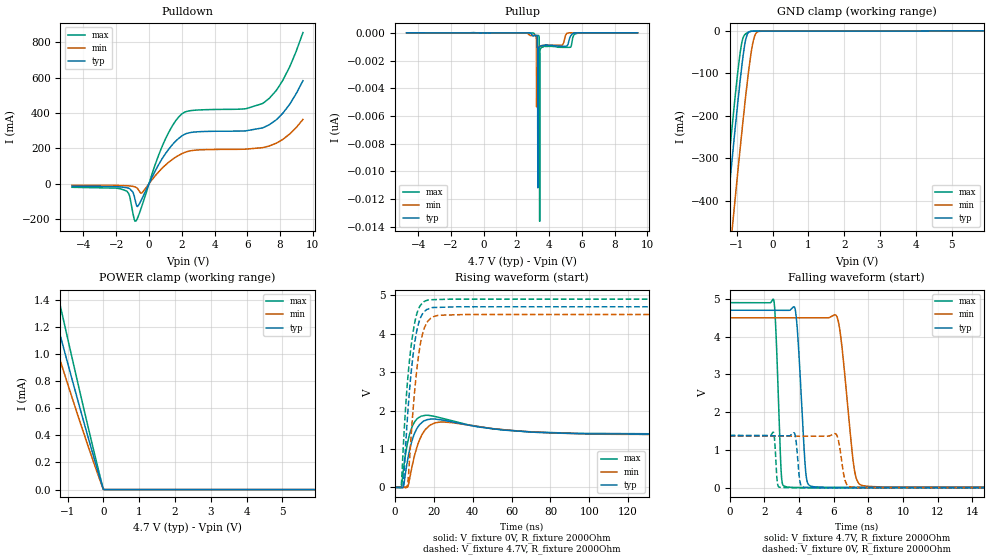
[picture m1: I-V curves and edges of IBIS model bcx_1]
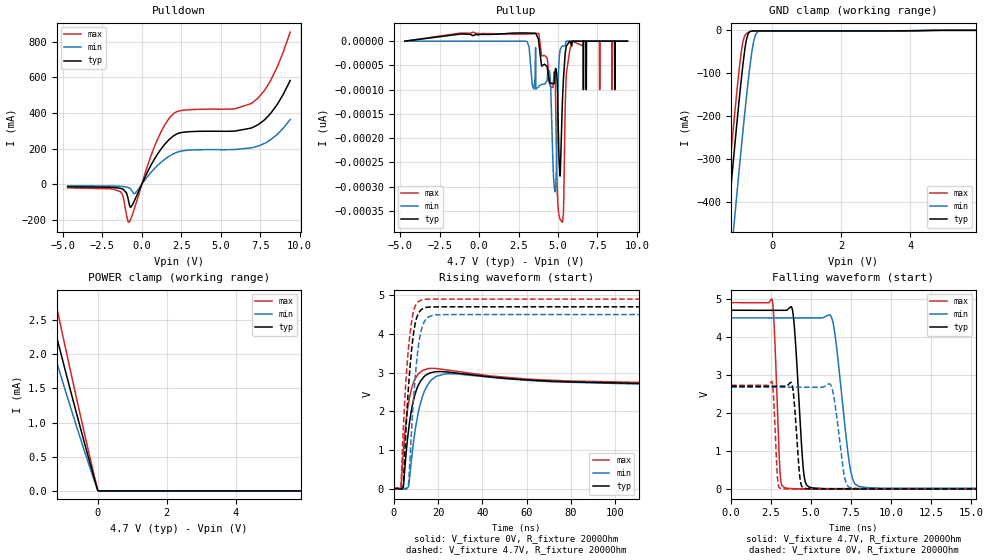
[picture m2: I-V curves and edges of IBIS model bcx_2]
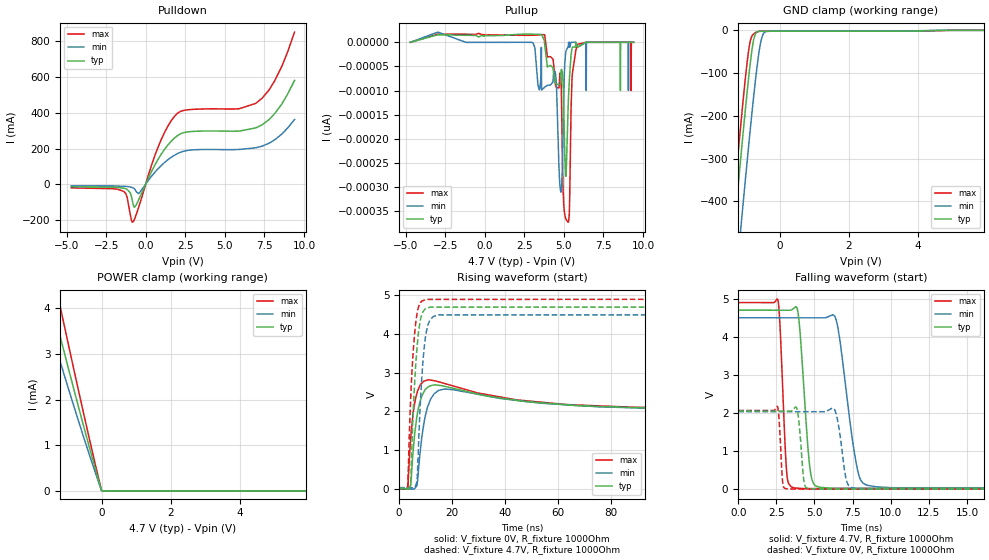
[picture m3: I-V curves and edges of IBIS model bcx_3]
| Texas Instruments Incorporated
| TPS546D24A- 2.95V to 16V, 40A, up to 4X stackable, PMBus(R) buck converter
| Marketing part#   Digital Voltage Range   Package-type   #pins
| TPS546D24A   0V - 5.5V   LQFN-CLIP   40
[IBIS Ver]   4.1
[File name]   tps546d24a.ibs
[File Rev]   1.0
[Date]   11/21/2019
[Source]
| Texas Instruments Incorporated.
| Analog-eLab Design Center, HPA
| 12500 TI Blvd
| Dallas, TX -75243
[Notes]   Revision History:
| Rev 1.0: 11/21/2019
| - Initial version of the model
| - Model generated from simulations in SPECTRE
| - C_comp although listed in numerical order of value are
|   obtained from varying PVT conditions. For PVT conditions for
|   each specific value refer the buffer description under
|   respective [Model]. IBIS model user is responsible for using
|   appropriate C_comp to simulate for Signal Integrity.
| - Warnings regarding combined Non-monotonicity of various models have been
|   reviewed and considered minor and can be ignored.
| - Model names with a trailing _1p8 contain the model for 1.8V operation.
|   Model names with a trailing _2p5 contain the model for 2.5V operation.
|   Model names with a trailing _3p3 contain the model for 3.3V operation.
|   Model names with a trailing _5p0 contain the model for 5.0V operation.
[Disclaimer]
| This model is designed as an aid for customers of Texas Instruments.
| TI and its licensors and suppliers make no warranties, either expressed
| or implied, with respect to this  model, including the warranties of
| merchantability or fitness for a particular purpose. The model is
| provided solely on an "as is" basis. The entire risk as to its quality
| and performance is with the customer.
| This model is subject to change without notice. Texas Instruments
| Incorporated is not responsible for updating this model
[Copyright]
(C) Copyright 2019 Texas Instruments Incorporated.All rights reserved.
|  Component TPS546D24RVF 40-Pin LQFN-CLIP -RVF package
|  Part # TPS546D24RVF
[Component]   TPS546D24RVF
[Manufacturer]   TI
[Package]   |40 LQFN-CLIP -RVF package
|   typ   min   max
R_pkg   0.05   0.04   0.06
L_pkg   1.0nH   0.8nH   1.2nH
C_pkg   0.2pF   0.16pF   0.24pF
[Pin] signal_name  model_name   R_pin   L_pin   C_pin
1   PGD/RST_B   pgd   NA   NA   NA
2   PMB_DATA   pmb   NA   NA   NA
3   PMB_CLK   pmb   NA   NA   NA
4   BP1V5   nc   NA   NA   NA
5   DRTN   nc   NA   NA   NA
6   SMB_ALRT   pmb   NA   NA   NA
7   BOOT   nc   NA   NA   NA
8   SW   nc   NA   NA   NA
9   SW   nc   NA   NA   NA
10   SW   nc   NA   NA   NA
11   SW   nc   NA   NA   NA
12   SW   nc   NA   NA   NA
13   PGND   gnd   NA   NA   NA
14   PGND   gnd   NA   NA   NA
15   PGND   gnd   NA   NA   NA
16   PGND   gnd   NA   NA   NA
17   PGND   gnd   NA   NA   NA
18   PGND   gnd   NA   NA   NA
19   PGND   gnd   NA   NA   NA
20   PGND   gnd   NA   NA   NA
21   PVIN   power   NA   NA   NA
22   PVIN   power   NA   NA   NA
23   PVIN   power   NA   NA   NA
24   PVIN   power   NA   NA   NA
25   PVIN   power   NA   NA   NA
26   AVIN   power   NA   NA   NA
27   EN/UVLO   nc   NA   NA   NA
28   VDD5   power   NA   NA   NA
29   MSEL2   nc   NA   NA   NA
30   VSEL   nc   NA   NA   NA
31   ADRSEL   nc   NA   NA   NA
32   MSEL1   nc   NA   NA   NA
33   VOSNS   nc   NA   NA   NA
34   GOSNS/SLAVE   nc   NA   NA   NA
35   VSHARE   nc   NA   NA   NA
36   NC   nc   NA   NA   NA
37   AGND   gnd   NA   NA   NA
38   SYNC   sync   NA   NA   NA
39   BCX_CLK   bcx   NA   NA   NA
40   BCX_DAT   bcx   NA   NA   NA
|   Model Selectors
[Model Selector] pmb
pmb_1p8   1.8V   Digital I/O
pmb_2p5   2.5V   Digital I/O
pmb_3p3   3.3V   Digital I/O
pmb_5p0   5.0V   Digital I/O
[Model Selector] bcx
bcx_1   One Pullup Current source block(672uA)   Digital I/O | 672uA constant pullup current
bcx_2   Two Pullup Current source blocks(2*672uA   Digital I/O | 1.34mA constant pullup current
bcx_3   Three Pullup Current source blocks(3*672uA)  Digital I/O | 2mA constant pullup current
| Models and submodels in the file (9): bcx_1 (I/O), bcx_2 (I/O), bcx_3 (I/O), pmb_1p8 (I/O_open_drain), pmb_2p5 (I/O_open_drain), pmb_3p3 (I/O_open_drain), pmb_5p0 (I/O_open_drain), pgd (I/O_open_drain), sync (I/O)
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|   bcx_1 Model
[Model]   bcx_1
Model_type   I/O
Polarity   Inverting
Enable   Active-High
Vinl = 0.8
Vinh = 1.35
Vmeas = 2.35
Vref = 0
Cref = 2pF
Rref = 100000
|   typ   min   max
C_comp   2.976pF   2.962pF   2.990pF
|C_comp_pull_up   2.976pF   2.962pF   2.990pF
|C_comp_pull_down   3.370pF   3.218pF   3.645pF
|  Where Nom  PVT is Nominal Process, 4.7V,  25C
|   Fast PVT is Strong Process,  4.9V,  -40C
|   Slow PVT is Weak Process,   4.5V,  150C
[Voltage Range]   4.7   4.5   4.9
|Junction Temperature
[Temperature Range]   25   150   -40
[Pullup Reference]   4.7   4.5   4.9
[Pulldown Reference]   0   0   0
[Power Clamp Reference]   4.7   4.5   4.9
[GND Clamp Reference]   0   0   0
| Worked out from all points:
|   slope of the pulldown table from 0 to 0.705 V, typ, clamps not added: 5.58 ohm
|   GND clamp passes 1 mA (typ) near -0.59 V on its own axis
|   POWER clamp passes 1 mA (typ) near -1.07 V on its own axis
|   falling waveform, V_fixture 4.7V, R_fixture 2000Ohm: 20-80 % time 340ps typ, 567ps min, 230ps max; typ from 4.7 V to 0.009 V
|   rising waveform, V_fixture 0V, R_fixture 2000Ohm: 20-80 % time 3.01ns typ, 3.88ns min, 2.35ns max; typ from 0 V to 1.38 V
|   rising waveform, V_fixture 4.7V, R_fixture 2000Ohm: 20-80 % time 4.82ns typ, 4.91ns min, 4.75ns max; typ from 0.009 V to 4.7 V
|   falling waveform, V_fixture 0V, R_fixture 2000Ohm: 20-80 % time 159ps typ, 276ps min, 104ps max; typ from 1.38 V to 0 V
[Pulldown]
|   Voltage   I(typ)   I(min)   I(max)
-4.7V     -13.03mA   -7.807mA   -19.31mA
-1.372V   -21.4mA    -10.46mA   -39.93mA
-1.175V   -27.33mA   -11.73mA   -70.85mA
-977.6mV  -47.06mA   -14.22mA   -167.8mA
-780.2mV  -116.5mA   -20.57mA   -208.3mA
-441.8mV  -86.15mA   -51.84mA   -127.7mA
799mV     141.5mA    88.06mA    211mA
1.786V    255.1mA    159.9mA    375.5mA
2.378V    287.2mA    183.7mA    411.3mA
7.003V    319.1mA    206.2mA    458.6mA
8.173V    399.9mA    251.8mA    586.2mA
9.4V      583.6mA    364.2mA    855.5mA
[GND Clamp]
|   Voltage   I(typ)   I(min)   I(max)
-4.7V     -3.614A    -3.753A    -3.556A
-1.415V   -552.2mA   -718.1mA   -475.4mA
-1.387V   -526.9mA   -693mA     -450mA
-1.358V   -501.7mA   -667.9mA   -424.6mA
-1.175V   -339.6mA   -506.1mA   -262.5mA
-1.076V   -254.6mA   -420.3mA   -178.5mA
-864.8mV  -85.71mA   -242.2mA   -29.58mA
-752mV    -20.4mA    -153.3mA   -6.976mA
-667.4mV  -3.13mA    -92.52mA   -2.572mA
-540.5mV  -779.1uA   -23.54mA   -798uA
-385.4mV  -692.5uA   -1.346mA   -696.8uA
9.4V      0A         0A         0A
[Pullup]
|   Voltage   I(typ)   I(min)   I(max)
-4.7V     0A         0A         0A
3.238V    -198.4pA   -5.351nA   -223.5pA
3.252V    -214.7pA   -1.335nA   -215.3pA
3.295V    -1.813nA   -1.09nA    -192.7pA
3.309V    -11.18nA   -1.068nA   -191.3pA
3.323V    -1.223nA   -1.048nA   -185.8pA
3.365V    -1.077nA   -1.002nA   -208.2pA
3.408V    -1.009nA   -972.6pA   -2.075nA
3.422V    -994.3pA   -965pA     -13.59nA
3.436V    -981.8pA   -958.2pA   -1.319nA
3.478V    -955.2pA   -942.1pA   -1.14nA
9.4V      0A         0A         0A
[POWER Clamp]
|   Voltage   I(typ)   I(min)   I(max)
-4.7V     4.841mA    4.462mA    5.649mA
-1.852V   1.785mA    1.503mA    2.128mA
-1.683V   1.613mA    1.356mA    1.924mA
-1.528V   1.457mA    1.223mA    1.739mA
-1.175V   1.106mA    925.7uA    1.321mA
-709.7mV  653.4uA    544.2uA    781.1uA
-314.9mV  282.1uA    233.9uA    337.5uA
-4.7mV    3.975uA    3.346uA    4.745uA
23.5mV    0A         0A         0A
9.4V      0A         0A         0A
[Ramp]
R_load = 2000
|   typ   min   max
dV/dt_r   0.827359/3.01437e-09   0.821238/3.8948e-09   0.83293/2.35068e-09
dV/dt_f   2.81451/3.39702e-10   2.69064/5.67144e-10   2.93668/2.30357e-10
[Falling Waveform]
V_fixture = 4.7V
V_fixture_min = 4.5V
V_fixture_max = 4.9V
R_fixture = 2000Ohm
C_fixture = 0F
|   Time   V(typ)   V(min)   V(max)
0s        4.7V       4.5V       4.9V
2.532ns   4.698V     4.499V     4.99V
3.009ns   4.698V     4.499V     209.5mV
3.791ns   4.697V     4.498V     9.359mV
4.45ns    212mV      4.498V     9.354mV
5.517ns   13.54mV    4.498V     9.346mV
6.303ns   13.53mV    4.331V     9.34mV
7.333ns   13.52mV    218.5mV    9.332mV
8.874ns   13.51mV    21.85mV    9.32mV
500ns     9.15mV     15.58mV    5.526mV
[Rising Waveform]
V_fixture = 0V
V_fixture_min = 0V
V_fixture_max = 0V
R_fixture = 2000Ohm
C_fixture = 0F
|   Time   V(typ)   V(min)   V(max)
0s        -2.427nV   5.037nV    271.9pV
3.238ns   656.8uV    388.6uV    -5.328mV
4.261ns   -190uV     511.4uV    444.5mV
6.531ns   731.8mV    13.27mV    1.18V
10ns      1.404V     824.6mV    1.699V
15.76ns   1.748V     1.516V     1.878V
24.37ns   1.754V     1.705V     1.798V
50.88ns   1.523V     1.527V     1.522V
91.31ns   1.404V     1.403V     1.41V
500ns     1.379V     1.369V     1.388V
[Rising Waveform]
V_fixture = 4.7V
V_fixture_min = 4.5V
V_fixture_max = 4.9V
R_fixture = 2000Ohm
C_fixture = 0F
|   Time   V(typ)   V(min)   V(max)
0s        9.15mV     15.58mV    5.526mV
3.185ns   9.792mV    10.32mV    27.19mV
4.261ns   67.08mV    8.545mV    1.075V
6.468ns   1.883V     67.45mV    2.788V
9.358ns   3.481V     2.076V     4.063V
11.85ns   4.221V     3.339V     4.619V
14.39ns   4.54V      4.041V     4.816V
17.2ns    4.647V     4.342V     4.879V
36.2ns    4.7V       4.5V       4.9V
500ns     4.7V       4.5V       4.9V
[Falling Waveform]
|Gnd
V_fixture = 0V
V_fixture_min = 0V
V_fixture_max = 0V
R_fixture = 2000Ohm
C_fixture = 0F
|   Time   V(typ)   V(min)   V(max)
0s        1.379V     1.369V     1.389V
2.523ns   1.377V     1.368V     1.474V
2.792ns   1.377V     1.368V     53.28mV
3.739ns   1.449V     1.367V     2.287mV
3.941ns   682.9mV    1.367V     1.025mV
4.174ns   33.24mV    1.367V     1.025mV
6.123ns   1.585mV    1.43V      1.021mV
6.773ns   1.583mV    82.23mV    1.02mV
8.526ns   1.577mV    2.589mV    1.016mV
500ns     -359.2pV   -5.119nV   309.4pV
|   bcx_2 Model
[Model]   bcx_2
Model_type   I/O
Polarity   Inverting
Enable   Active-High
Vinl = 0.8
Vinh = 1.35
Vmeas = 2.35
Vref = 0
Cref = 2pF
Rref = 100000
|   typ   min   max
C_comp   2.976pF   2.976pF   2.990pF
|C_comp_pull_up   2.976pF   2.962pF   2.977pF
|C_comp_pull_down   3.204pF   3.088pF   3.401pF
|  Where Nom  PVT is Nominal Process, 4.7V,  25C
|   Fast PVT is Strong Process,  4.9V,  -40C
|   Slow PVT is Weak Process,   4.5V,  150C
[Voltage Range]   4.7   4.5   4.9
|Junction Temperature
[Temperature Range]   25   150   -40
[Pullup Reference]   4.7   4.5   4.9
[Pulldown Reference]   0   0   0
[Power Clamp Reference]   4.7   4.5   4.9
[GND Clamp Reference]   0   0   0
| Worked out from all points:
|   slope of the pulldown table from 0 to 0.705 V, typ, clamps not added: 5.58 ohm
|   POWER clamp passes 1 mA (typ) near -0.55 V on its own axis
|   falling waveform, V_fixture 4.7V, R_fixture 2000Ohm: 20-80 % time 398ps typ, 688ps min, 264ps max; typ from 4.7 V to 0.009 V
|   rising waveform, V_fixture 0V, R_fixture 2000Ohm: 20-80 % time 3.4ns typ, 4.17ns min, 2.75ns max; typ from 0 V to 2.71 V
|   rising waveform, V_fixture 4.7V, R_fixture 2000Ohm: 20-80 % time 3.38ns typ, 3.49ns min, 3.27ns max; typ from 0.009 V to 4.7 V
|   falling waveform, V_fixture 0V, R_fixture 2000Ohm: 20-80 % time 278ps typ, 479ps min, 180ps max; typ from 2.71 V to 0 V
[Pulldown]
|   Voltage   I(typ)   I(min)   I(max)
-4.7V     -12.99mA   -7.762mA   -19.27mA
-1.372V   -21.32mA   -10.38mA   -39.86mA
-1.175V   -27.24mA   -11.64mA   -70.76mA
-977.6mV  -46.92mA   -14.12mA   -167.7mA
-780.2mV  -116.1mA   -20.42mA   -207.7mA
-441.8mV  -85.46mA   -51.2mA    -127mA
799mV     142.2mA    88.74mA    211.7mA
1.786V    255.8mA    160.6mA    376.2mA
2.576V    291.6mA    188.3mA    415.1mA
7.003V    318.3mA    205.9mA    457.3mA
8.173V    398.9mA    251.3mA    584.4mA
9.4V      582mA      363.3mA    852.9mA
[GND Clamp]
|   Voltage   I(typ)   I(min)   I(max)
-4.7V     -3.614A    -3.753A    -3.556A
-1.415V   -552.3mA   -718.2mA   -475.5mA
-1.387V   -527mA     -693mA     -450mA
-1.358V   -501.7mA   -667.9mA   -424.7mA
-1.175V   -339.7mA   -506.2mA   -262.6mA
-1.076V   -254.7mA   -420.4mA   -178.6mA
-864.8mV  -85.91mA   -242.3mA   -29.97mA
-766.1mV  -26.69mA   -164.2mA   -8.741mA
-667.4mV  -3.776mA   -92.75mA   -3.245mA
-540.5mV  -1.469mA   -23.98mA   -1.492mA
-385.4mV  -1.384mA   -2.021mA   -1.393mA
9.4V      0A         0A         0A
[Pullup]
|   Voltage   I(typ)   I(min)   I(max)
-4.7V     0A         0A         0A
3.788V    -5pA       -92.8pA    14.9pA
4.451V    -83.2pA    -60.9pA    -84.9pA
4.817V    -62.2pA    -310.8pA   -82.8pA
4.958V    -95.3pA    -162.3pA   -315.9pA
5.128V    -278.2pA   -20pA      -366.9pA
5.255V    -148.2pA   -10pA      -373.2pA
5.508V    -13pA      0A         -79.2pA
5.889V    0A         0A         0A
6.608V    -100pA     0A         0A
7.638V    0A         0A         -100pA
9.4V      0A         0A         0A
[POWER Clamp]
|   Voltage   I(typ)   I(min)   I(max)
-4.7V     9.671mA    8.914mA    11.28mA
-1.852V   3.566mA    3.004mA    4.25mA
-1.697V   3.252mA    2.735mA    3.878mA
-1.499V   2.855mA    2.396mA    3.406mA
-1.175V   2.211mA    1.85mA     2.64mA
-766.1mV  1.414mA    1.178mA    1.69mA
-371.3mV  667.9uA    554.2uA    798.7uA
-4.7mV    8.089uA    6.692uA    9.665uA
23.5mV    0A         0A         0A
9.4V      0A         0A         0A
[Ramp]
R_load = 2000
|   typ   min   max
dV/dt_r   1.62317/3.40511e-09   1.60666/4.16841e-09   1.63751/2.75863e-09
dV/dt_f   2.81451/3.97943e-10   2.69064/6.88264e-10   2.93668/2.64301e-10
[Falling Waveform]
V_fixture = 4.7V
V_fixture_min = 4.5V
V_fixture_max = 4.9V
R_fixture = 2000Ohm
C_fixture = 0F
|   Time   V(typ)   V(min)   V(max)
0s        4.7V       4.5V       4.9V
2.56ns    4.698V     4.499V     4.989V
3.119ns   4.698V     4.499V     196mV
3.79ns    4.777V     4.499V     14.95mV
4.035ns   3.817V     4.498V     9.15mV
4.698ns   133mV      4.498V     9.145mV
6.299ns   13.29mV    4.496V     9.134mV
7.657ns   13.28mV    210.8mV    9.124mV
9.53ns    13.27mV    20.93mV    9.11mV
500ns     9.15mV     15.58mV    5.526mV
[Rising Waveform]
V_fixture = 0V
V_fixture_min = 0V
V_fixture_max = 0V
R_fixture = 2000Ohm
C_fixture = 0F
|   Time   V(typ)   V(min)   V(max)
0s        -6.173nV   232pV      -228.1pV
3.229ns   -9.546mV   -5.91mV    24.76mV
4.326ns   53.39mV    -7.921mV   969.3mV
6.62ns    1.491V     55.89mV    2.2V
8.404ns   2.163V     969.4mV    2.66V
11ns      2.667V     1.956V     2.962V
15.46ns   2.965V     2.695V     3.103V
24.68ns   3.012V     2.972V     3.063V
109ns     2.725V     2.707V     2.75V
500ns     2.705V     2.678V     2.729V
[Rising Waveform]
V_fixture = 4.7V
V_fixture_min = 4.5V
V_fixture_max = 4.9V
R_fixture = 2000Ohm
C_fixture = 0F
|   Time   V(typ)   V(min)   V(max)
0s        9.15mV     15.58mV    5.526mV
3.214ns   9.757mV    10.61mV    48.23mV
4.326ns   116.9mV    8.884mV    1.582V
6.559ns   2.561V     100.2mV    3.585V
8.404ns   3.78V      1.874V     4.448V
10ns      4.351V     3.098V     4.761V
11.45ns   4.559V     3.818V     4.849V
13.25ns   4.655V     4.252V     4.888V
24.68ns   4.7V       4.5V       4.9V
500ns     4.7V       4.5V       4.9V
[Falling Waveform]
|Gnd
V_fixture = 0V
V_fixture_min = 0V
V_fixture_max = 0V
R_fixture = 2000Ohm
C_fixture = 0F
|   Time   V(typ)   V(min)   V(max)
0s        2.705V     2.678V     2.729V
2.545ns   2.704V     2.677V     2.83V
2.959ns   2.703V     2.677V     100.4mV
3.917ns   2.436V     2.676V     2.259mV
4.275ns   423.8mV    2.676V     2.257mV
4.464ns   48.14mV    2.676V     2.257mV
6.201ns   3.489mV    2.756V     2.249mV
7.23ns    3.482mV    131.6mV    2.244mV
8.973ns   3.47mV     3.468mV    2.236mV
500ns     -610.1pV   7.057nV    1.367nV
|   bcx_3 Model
[Model]   bcx_3
Model_type   I/O
Polarity   Inverting
Enable   Active-High
Vinl = 0.8
Vinh = 1.35
Vmeas = 2.35
Vref = 0
Cref = 2pF
Rref = 100000
|   typ   min   max
C_comp   2.990pF   2.976pF   2.990pF
|C_comp_pull_up   2.977pF   2.976pF   2.990pF
|C_comp_pull_down   3.189pF   3.116pF   3.324pF
|  Where Nom  PVT is Nominal Process, 4.7V,  25C
|   Fast PVT is Strong Process,  4.9V,  -40C
|   Slow PVT is Weak Process,   4.5V,  150C
[Voltage Range]   4.7   4.5   4.9
|Junction Temperature
[Temperature Range]   25   150   -40
[Pullup Reference]   4.7   4.5   4.9
[Pulldown Reference]   -0   0   0
[Power Clamp Reference]   4.7   4.5   4.9
[GND Clamp Reference]   0   0   0
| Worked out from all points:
|   slope of the pulldown table from 0 to 0.705 V, typ, clamps not added: 5.58 ohm
|   POWER clamp passes 1 mA (typ) near -0.37 V on its own axis
|   falling waveform, V_fixture 4.7V, R_fixture 1000Ohm: 20-80 % time 481ps typ, 864ps min, 310ps max; typ from 4.7 V to 0.018 V
|   rising waveform, V_fixture 0V, R_fixture 1000Ohm: 20-80 % time 1.58ns typ, 2ns min, 1.25ns max; typ from 0 V to 2.05 V
|   rising waveform, V_fixture 4.7V, R_fixture 1000Ohm: 20-80 % time 2.15ns typ, 2.2ns min, 2.09ns max; typ from 0.018 V to 4.7 V
|   falling waveform, V_fixture 0V, R_fixture 1000Ohm: 20-80 % time 242ps typ, 412ps min, 163ps max; typ from 2.05 V to 0 V
[Pulldown]
|   Voltage   I(typ)   I(min)   I(max)
-4.7V     -12.95mA   -7.717mA   -19.24mA
-1.372V   -21.25mA   -10.31mA   -39.79mA
-1.175V   -27.15mA   -11.56mA   -70.67mA
-977.6mV  -46.79mA   -14.01mA   -167.5mA
-780.2mV  -115.8mA   -20.26mA   -207.1mA
-441.8mV  -84.77mA   -50.56mA   -126.4mA
799mV     142.9mA    89.43mA    212.4mA
1.786V    256.5mA    161.3mA    376.9mA
2.576V    292.3mA    189mA      415.8mA
7.003V    317.4mA    205.5mA    456mA
8.173V    397.9mA    250.8mA    582.7mA
9.4V      580.5mA    362.3mA    850.4mA
[GND Clamp]
|   Voltage   I(typ)   I(min)   I(max)
-4.7V     -3.614A    -3.753A    -3.556A
-1.415V   -552.4mA   -718.3mA   -475.5mA
-1.387V   -527.1mA   -693.1mA   -450.1mA
-1.358V   -501.8mA   -668mA     -424.8mA
-1.175V   -339.8mA   -506.3mA   -262.7mA
-1.076V   -254.8mA   -420.5mA   -178.8mA
-864.8mV  -86.11mA   -242.5mA   -30.37mA
-766.1mV  -27.07mA   -164.3mA   -9.378mA
-667.4mV  -4.424mA   -92.98mA   -3.919mA
-540.5mV  -2.159mA   -24.42mA   -2.187mA
-385.4mV  -2.076mA   -2.696mA   -2.089mA
9.4V      0A         0A         0A
[Pullup]
|   Voltage   I(typ)   I(min)   I(max)
-4.7V     0A         0A         0A
3.788V    -4.9pA     -92.9pA    15pA
4.451V    -83.2pA    -60.8pA    -84.8pA
4.817V    -62.6pA    -310.9pA   -82.3pA
5.114V    -276.8pA   -23pA      -365.6pA
5.255V    -149pA     -10pA      -373.2pA
5.508V    -13pA      0A         -79.6pA
5.875V    -10pA      -10pA      -4pA
9.076V    0A         -100pA     0A
9.231V    0A         0A         0A
9.245V    0A         0A         -100pA
9.4V      0A         0A         0A
[POWER Clamp]
|   Voltage   I(typ)   I(min)   I(max)
-4.7V     14.49mA    13.36mA    16.91mA
-1.852V   5.343mA    4.502mA    6.368mA
-1.697V   4.873mA    4.098mA    5.81mA
-1.499V   4.279mA    3.591mA    5.104mA
-1.175V   3.313mA    2.773mA    3.955mA
-766.1mV  2.119mA    1.766mA    2.532mA
-371.3mV  1.001mA    830.7uA    1.197mA
-4.7mV    12.14uA    10.04uA    14.5uA
23.5mV    0A         0A         0A
9.4V      0A         0A         0A
[Ramp]
R_load = 1000
|   typ   min   max
dV/dt_r   1.23105/1.55331e-09   1.22133/1.97471e-09   1.24019/1.23377e-09
dV/dt_f   2.80901/4.80255e-10   2.68131/8.62896e-10   2.93336/3.09838e-10
[Falling Waveform]
V_fixture = 4.7V
V_fixture_min = 4.5V
V_fixture_max = 4.9V
R_fixture = 1000Ohm
C_fixture = 0F
|   Time   V(typ)   V(min)   V(max)
0s        4.7V       4.5V       4.9V
2.59ns    4.698V     4.499V     4.985V
3.216ns   4.698V     4.499V     300.6mV
3.882ns   4.721V     4.499V     26.7mV
4.299ns   2.69V      4.499V     14.75mV
5.019ns   105.5mV    4.498V     14.74mV
6.417ns   22.95mV    4.45V      14.73mV
7.989ns   22.93mV    276mV      14.72mV
10.1ns    22.91mV    38.25mV    14.71mV
500ns     18.31mV    31.17mV    11.06mV
[Rising Waveform]
V_fixture = 0V
V_fixture_min = 0V
V_fixture_max = 0V
R_fixture = 1000Ohm
C_fixture = 0F
|   Time   V(typ)   V(min)   V(max)
0s        -3.462nV   878.6pV    -657.8pV
3.216ns   -9.265mV   -5.615mV   30.07mV
4.28ns    46.61mV    -7.472mV   1.233V
5.249ns   949.8mV    -9.163mV   1.935V
6.637ns   1.837V     73.14mV    2.445V
8.697ns   2.415V     1.408V     2.738V
10.95ns   2.63V      2.152V     2.814V
17.4ns    2.642V     2.577V     2.715V
89.05ns   2.096V     2.091V     2.105V
500ns     2.052V     2.036V     2.067V
[Rising Waveform]
V_fixture = 4.7V
V_fixture_min = 4.5V
V_fixture_max = 4.9V
R_fixture = 1000Ohm
C_fixture = 0F
|   Time   V(typ)   V(min)   V(max)
0s        18.31mV    31.17mV    11.06mV
3.216ns   10.06mV    27.05mV    67.77mV
4.28ns    108.1mV    25.69mV    2.235V
5.38ns    2.103V     24.29mV    3.617V
6.637ns   3.555V     174.1mV    4.477V
8.482ns   4.482V     2.8V       4.844V
10.15ns   4.651V     4.01V      4.891V
11.7ns    4.69V      4.362V     4.891V
14.8ns    4.69V      4.489V     4.891V
500ns     4.7V       4.5V       4.9V
[Falling Waveform]
|Gnd
V_fixture = 0V
V_fixture_min = 0V
V_fixture_max = 0V
R_fixture = 1000Ohm
C_fixture = 0F
|   Time   V(typ)   V(min)   V(max)
0s        2.052V     2.036V     2.067V
2.571ns   2.05V      2.035V     2.17V
2.952ns   2.05V      2.035V     86.32mV
3.821ns   2.144V     2.034V     3.683mV
4.043ns   1.501V     2.034V     1.93mV
4.469ns   38.37mV    2.034V     1.928mV
6.253ns   2.67mV     2.12V      1.921mV
7.178ns   2.665mV    138.5mV    1.917mV
9.197ns   2.655mV    3.034mV    1.91mV
500ns     -1.678nV   -8.061nV   -7.001nV
